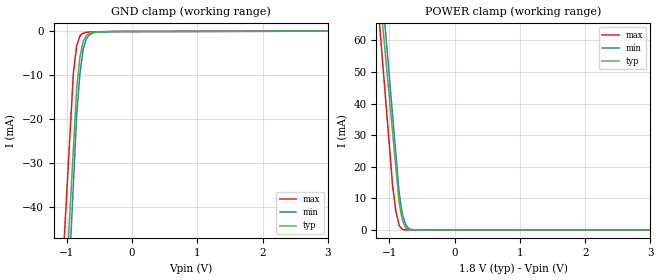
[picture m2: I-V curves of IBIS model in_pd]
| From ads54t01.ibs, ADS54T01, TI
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[Model] in_pd
Model_type Input
Vinl = 540.000mV
Vinh = 1.26000V
C_comp 722.000fF 722.000fF 722.000fF
| variable typ   min   max
[Voltage Range] 1.80000V 1.65000V 1.95000V
[POWER Clamp Reference] 1.80000V 1.65000V 1.95000V
[GND Clamp Reference] 0.00000V 0.00000V 0.00000V
[Temperature Range]   25   85   -40
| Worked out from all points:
|   GND clamp passes 1 mA (typ) near -0.70 V on its own axis
|   POWER clamp passes 1 mA (typ) near -0.76 V on its own axis
[GND Clamp]
-1.8V     -273.5mA   -316.5mA   -250.6mA
-900mV    -26.74mA   -34.8mA    -9.459mA
-850mV    -13.03mA   -19.15mA   -3.209mA
-800mV    -5.805mA   -9.644mA   -1.012mA
-750mV    -2.213mA   -4.068mA   -392.2uA
-700mV    -875.4uA   -1.626mA   -195.3uA
-650mV    -414.1uA   -743.4uA   -120.2uA
-550mV    -169.3uA   -163.1uA   -86.49uA
3.6V      79.9uA     85.29uA    71.29uA
[POWER Clamp]
-1.8V     219.9mA    243.6mA    231.6mA
-1.1V     64.19mA    72.82mA    52.24mA
-1.05V    53.07mA    60.62mA    39.42mA
-950mV    30.82mA    36.21mA    13.8mA
-900mV    19.69mA    24.01mA    5.892mA
-850mV    8.567mA    11.81mA    1.376mA
-800mV    3.024mA    4.892mA    178uA
-750mV    693.8uA    1.664mA    17.27uA
-700mV    119.3uA    360.9uA    15.35uA
-650mV    102.2uA    67.51uA    13.43uA
3.6V      0A         0A         0A
